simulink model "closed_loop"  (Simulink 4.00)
settings: Solver=ode45  StartTime=0.0  StopTime=10.0  RelTol=1e-3
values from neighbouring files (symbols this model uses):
  Amp = 1    [EXAMPLE1.M]    (also in EXAMPLE2.M; EXAMPLE3.M)
  omega = 6    [EXAMPLE1.M]    (also in EXAMPLE2.M = 0; EXAMPLE3.M = 0)
  t0 = 1    [EXAMPLE1.M]    (also in EXAMPLE2.M; EXAMPLE3.M)
  u0 = 1    [EXAMPLE1.M]    (also in EXAMPLE2.M; EXAMPLE3.M)
libraries: cstblocks x2

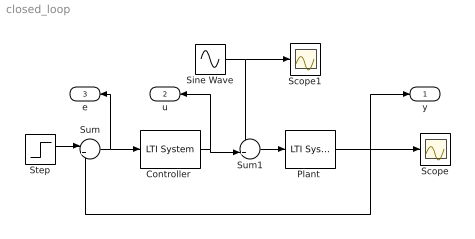
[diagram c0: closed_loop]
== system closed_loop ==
  "Controller " : cstblocks/LTI System  sys=C  IC=[]
  "Plant " : cstblocks/LTI System  sys=Go  IC=[]
  Scope : Scope
  Scope1 : Scope
  Sine Wave : Sin  SineType=Time-based  Amplitude=Amp  Bias=0  Frequency=omega  Phase=0  Samples=10  SampleTime=0
  Step : Step  Time=t0  Before=0  After=u0  SampleTime=0
  Sum : Sum  Inputs=|+-  SaturateOnIntegerOverflow=on
  Sum1 : Sum  Inputs=++|  SaturateOnIntegerOverflow=on
  y : Outport  Port=1
  u : Outport  Orientation=left  Port=2
  e : Outport  Orientation=left  Port=3
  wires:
  "Controller "/1 -> Sum1/2, u/1
  Sum1/1 -> "Plant "/1
  "Plant "/1 -> Scope/1, Sum/2, y/1
  Sum/1 -> "Controller "/1, e/1
  Step/1 -> Sum/1
  Sine Wave/1 -> Sum1/1, Scope1/1
